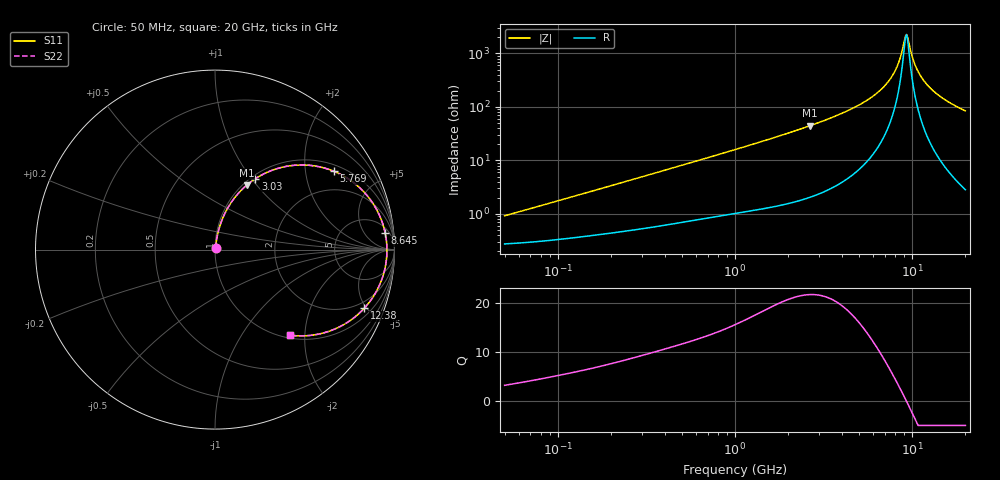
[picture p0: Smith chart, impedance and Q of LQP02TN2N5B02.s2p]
!Murata Part Number: LQP02TN2N5B02
!These Parameters are Measured in Series Mode Connection
!  o--[Z]--o
!Port1  Port2
!  o-------o
!Freq. Start=50[MHz] Stop=20[GHz], 401[Steps]
# Hz S RI R 50
!Freq.(Hz) S11(Real) S11(Imag) S21(Real) S21(Imag) S12(Real) S12(Imag) S22(Real) S22(Imag)
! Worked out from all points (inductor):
!   401 points, 50 MHz to 20 GHz, reference 50 ohm
!   read as one part in series: L = 2.79 nH near 51.52 MHz
!   highest Q = 21.8 at 2.647 GHz (marker M1), where L = 2.67 nH
!   self-resonance near 9.284 GHz
!   S11 on the Smith chart (normalised r, x): 50 MHz: 1.01, +0.02; 3.03 GHz: 1.05, +1.04; 5.769 GHz: 1.22, +2.88; 8.645 GHz: 8, +17; 12.38 GHz: 1.49, -4.84; 20 GHz: 1.06, -1.69
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5e7  0.00282 0.00877  0.9972 -0.00877  0.9972 -0.00877  0.00282 0.00877
1.364002e8  0.00425 0.0231  0.9957 -0.0231  0.9957 -0.0231  0.00425 0.0231
3.721004e8  0.00949 0.0598  0.9905 -0.0598  0.9905 -0.0598  0.00949 0.0598
1e9  0.034 0.152  0.966 -0.152  0.966 -0.152  0.034 0.152
1.740566e9  0.0836 0.2528  0.9164 -0.2528  0.9164 -0.2528  0.0836 0.2528
2.647493e9  0.1763 0.3588  0.8237 -0.3588  0.8237 -0.3588  0.1763 0.3588
2.728004e9  0.1861 0.3669  0.8139 -0.3669  0.8139 -0.3669  0.1861 0.3669
3.029571e9  0.2251 0.3952  0.7749 -0.3952  0.7749 -0.3952  0.2251 0.3952
4.472136e9  0.448 0.4703  0.552 -0.4703  0.552 -0.4703  0.448 0.4703
5.769027e9  0.6637 0.4359  0.3363 -0.4359  0.3363 -0.4359  0.6637 0.4359
6.601595e9  0.7842 0.3638  0.2158 -0.3638  0.2158 -0.3638  0.7842 0.3638
7.442007e9  0.877 0.2617  0.123 -0.2617  0.123 -0.2617  0.877 0.2617
8.141811e9  0.9275 0.1638  0.0725 -0.1638  0.0725 -0.1638  0.9275 0.1638
8.644534e9  0.9484 0.0911  0.0516 -0.0911  0.0516 -0.0911  0.9484 0.0911
9.041845e9  0.9564 0.0342  0.0436 -0.0342  0.0436 -0.0342  0.9564 0.0342
9.316812e9  0.9579 -0.00418  0.0421 0.00418  0.0421 0.00418  0.9579 -0.00418
9.457416e9  0.9575 -0.0234  0.0425 0.0234  0.0425 0.0234  0.9575 -0.0234
1.019291e10  0.944 -0.1181  0.056 0.1181  0.056 0.1181  0.944 -0.1181
1.066139e10  0.927 -0.1724  0.073 0.1724  0.073 0.1724  0.927 -0.1724
1.238412e10  0.8321 -0.3264  0.1679 0.3264  0.1679 0.3264  0.8321 -0.3264
1.527346e10  0.6465 -0.451  0.3535 0.451  0.3535 0.451  0.6465 -0.451
2e10  0.4193 -0.477  0.5807 0.477  0.5807 0.477  0.4193 -0.477
